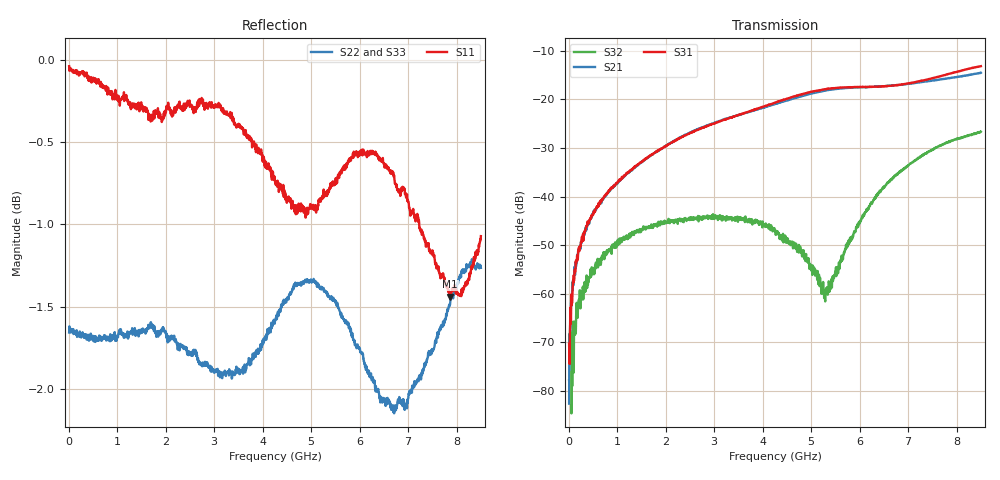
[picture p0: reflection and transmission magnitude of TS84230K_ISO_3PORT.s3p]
! Created with skrf (http://scikit-rf.org).
# Hz S RI R 50.0
!freq ReS11 ImS11 ReS12 ImS12 ReS13 ImS13
! ReS21 ImS21 ReS22 ImS22 ReS23 ImS23
! ReS31 ImS31 ReS32 ImS32 ReS33 ImS33
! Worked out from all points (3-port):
!   1601 points, 10 MHz to 8.5 GHz, reference 50 ohm
!   strongest paths, dB at 10 MHz, 2.132 GHz, 4.255 GHz, 6.378 GHz, 8.5 GHz:
!     S31: -70.3, -28.9, -20.7, -17.4, -13.2
!     S21: -82.6, -28.9, -21.0, -17.4, -14.5
!     S32: -77.9, -44.9, -47.1, -39.7, -26.7
!   lowest |S11| = -1.4 dB at 7.869 GHz (marker M1), VSWR 12.10, Z = 4.29 + j9.6 ohm
!   |S11| at or under -10 dB: nowhere
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1e7  0.9957 -0.00684  5.57e-05 7.11e-05  0.000308 0.000216
     5.87e-05 4.48e-05  -0.8263 0.00474  0.000139 8.06e-05
     8e-05 0.000294  0.000127 4.01e-06  -0.8234 0.00515
7.898125e7  0.9912 -0.0366  7.64e-05 0.000975  0.000284 0.00124
            0.000245 0.00127  -0.8269 0.031  -0.000115 0.000405
            0.000373 0.000985  3.15e-05 0.000164  -0.8229 0.027
1.798e8  0.9882 -0.0846  0.000441 0.00238  0.000164 0.00229
         0.000192 0.00251  -0.8223 0.0687  0.000159 0.000674
         0.000199 0.00219  -0.000116 0.000638  -0.8202 0.0638
7.634875e8  0.9206 -0.3376  0.000231 0.0104  0.000212 0.0107
            0.000378 0.0103  -0.7772 0.2704  0.00107 0.00231
            3.66e-05 0.0104  0.000818 0.00242  -0.7807 0.2562
2.689656e9  0.2143 -0.9444  0.015 0.0475  0.0144 0.047
            0.0149 0.0472  -0.4392 0.6794  0.00483 0.00363
            0.0141 0.0471  0.00468 0.0037  -0.4699 0.6673
4.255e9  -0.3569 -0.8464  0.059 0.0674  0.0574 0.0724
         0.0586 0.0675  0.0582 0.8315  0.00396 0.000911
         0.0575 0.0725  0.00434 0.000751  -0.0521 0.8226
5.310944e9  -0.7703 -0.4856  0.1102 0.0563  0.1128 0.0598
            0.1099 0.0561  0.2971 0.7969  -0.00012 0.000929
            0.1123 0.0598  2.09e-05 0.00114  0.2739 0.7998
6.3775e9  -0.9312 0.0777  0.1348 0.0128  0.1338 0.0199
          0.1348 0.013  0.4247 0.6705  -0.00838 0.00643
          0.1339 0.0198  -0.00829 0.00627  0.345 0.7449
7.868556e9  -0.7862 0.316  0.1598 -0.0455  0.1827 -0.0257
            0.1596 -0.045  0.7873 0.3036  -0.00547 0.0369
            0.1827 -0.0253  -0.00548 0.0369  0.6266 0.5164
8.5e9  -0.7077 0.5298  0.1663 -0.087  0.2036 -0.0845
       0.1667 -0.0862  0.8505 0.1556  0.00823 0.0458
       0.2032 -0.0832  0.00721 0.0458  0.7869 0.3125
